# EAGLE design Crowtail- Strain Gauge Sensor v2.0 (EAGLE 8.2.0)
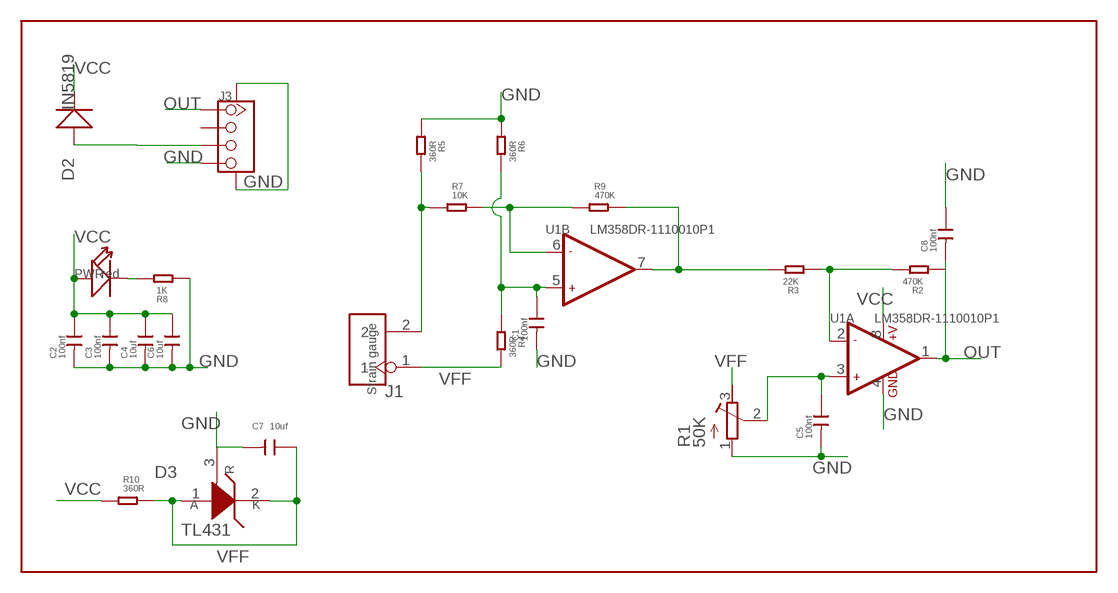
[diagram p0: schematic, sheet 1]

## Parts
C1  100nf  C-0603  [C0603]
C2  100nf  C-0603  [C0603]
C3  100nf  C-0603  [C0603]
C4  10uf  C-0603  [C0603]
C5  100nf  C-0603  [C0603]
C6  10uf  C-0603  [C0603]
C7  10uf  C-0603  [C0603]
C8  100nf  C-0603  [C0603]
D2  IN5819  D'0805'  [SOD323]
D3  TL431  [SOT23]
J1  Strain gauge  HEADER-2P-65/35MIL  [2P-2.54-65/35MIL]
J3  TWIG-4P-2.0-SMD-FEMALE-REINFORCE'90D'  [4P-SMD-2.0-90D]
PWR  red  LED'0603'  [LED-0603]
R1  50K  R-TRIMM3296P  [RTRIM3296P]
R2  470K  R-0603  [R0603]
R3  22K  R-0603  [R0603]
R4  360R  R-0603  [R0603]
R5  360R  R-0603  [R0603]
R6  360R  R-0603  [R0603]
R7  10K  R-0603  [R0603]
R8  1K  R-0603  [R0603]
R9  470K  R-0603  [R0603]
R10  360R  R-0603  [R0603]
U1  LM358DR-1110010P1  [SOIC8]

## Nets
GND: C1.2 C2.2 C3.2 C4.2 C5.2 C6.2 C7.2 C8.1 D3.3(R) J3.4 J3.SS1 J3.SS2 R1.1(E) R5.1 R6.1 R8.1 U1.4(A:GND)
N$1: C5.1 R1.2(S) U1.3(A:+IN1)
N$2: R2.2 R3.1 U1.2(A:-IN1)
N$3: R3.2 R9.2 U1.7(B:OUT2)
N$5: R7.2 R9.1 U1.6(B:-IN2)
N$6: J1.2 R5.2 R7.1
N$7: C1.1 R4.1 R6.2 U1.5(B:+IN2)
N$8: PWR.- R8.2
N$9: D2.+ J3.3
OUT: C8.2 J3.1 R2.1 U1.1(A:OUT1)
VCC: C2.1 C3.1 C4.1 C6.1 D2.- PWR.+ R10.1 U1.8(A:+V)
VFF: C7.1 D3.1(A) D3.2(K) J1.1 R1.3(A) R4.2 R10.2
Unconnected: J3.2

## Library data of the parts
C1-C8 = Discrete:C*: Ceramic Capacitors
D2 = Discrete:D*
D3 = Discrete:TL431
J1 = Connector:HEADER-2P
J3 = Connector:TWIG-4P-2.0-SMD-FEMALE-REINFORCE
PWR = Discrete:LED*
R1 = resistor:R-TRIMM: Trimm resistor
R2-R10 = Discrete:R*
U1 = OPL Eagle Library:LM358DR: General purpose LOW Voltage, Rail-to-Rail Output Amplifiers http://www.fairchildsemi.com/ds/LM/LMV358.pdf

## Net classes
3 usbvcc: width 0.203 mm, drill 0.305 mm, clearance 0.203 mm

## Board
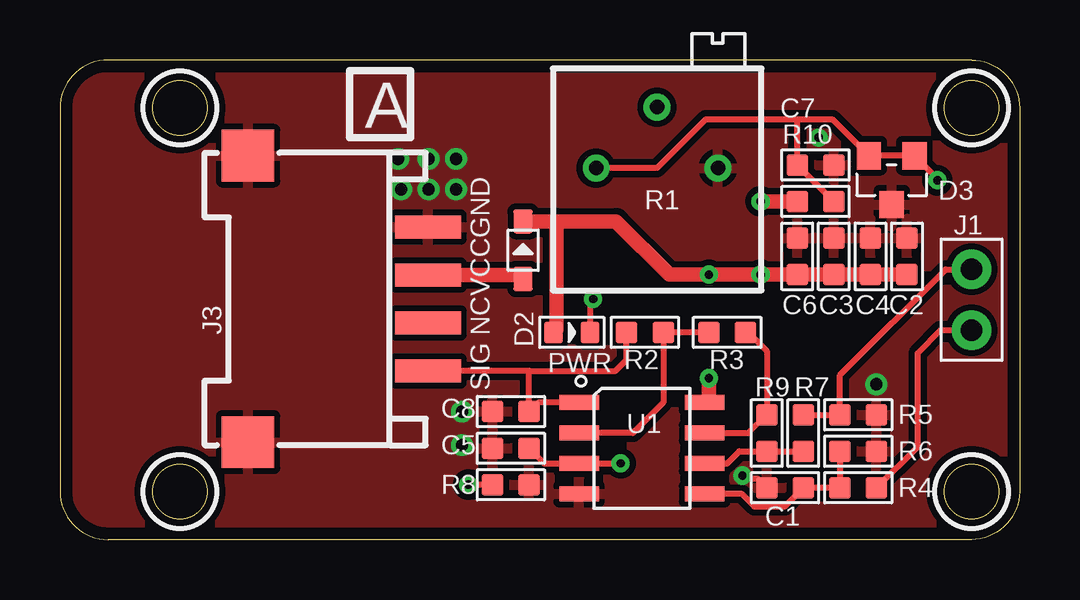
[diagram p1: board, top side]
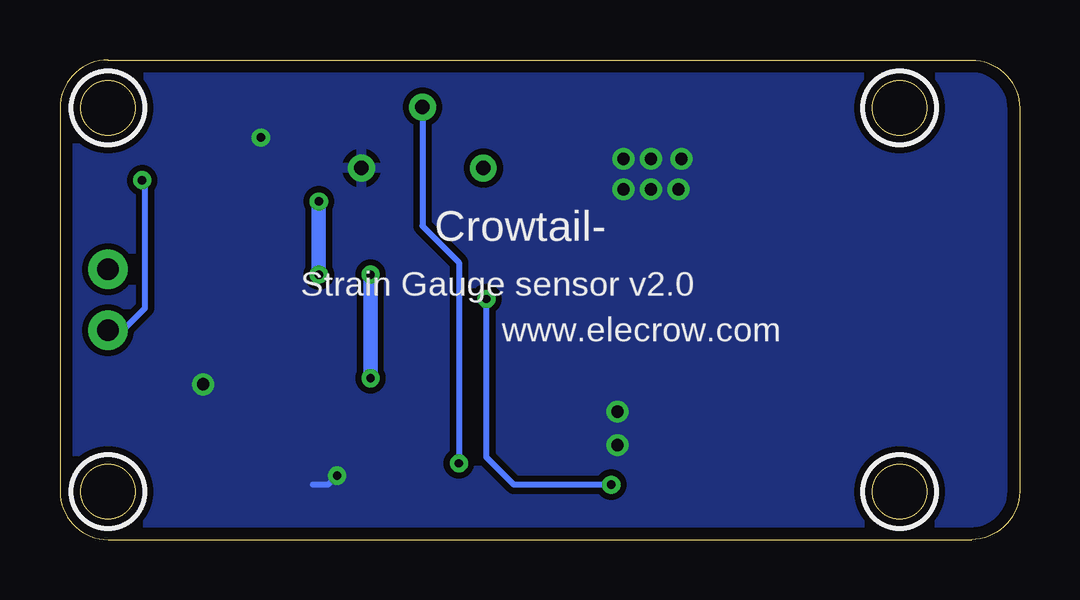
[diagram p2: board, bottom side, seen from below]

Size 40 x 20 mm. Coordinates in mm from the lower left corner, seen from the top.
Outline: 38,20 2,20 arc90 0,18 0,2 arc90 2,0 38,0 arc90 40,2 40,18 arc90 38,20
Outline: circle at 5,18 radius 1.14
Outline: circle at 5,2 radius 1.14
Outline: circle at 38,18 radius 1.14
Outline: circle at 38,2 radius 1.14
Copper layers (1*16): Top 0.035mm / dielectric 1.5mm / Bottom 0.035mm
Design rules "default *": minimum track width 10mil, minimum drill 20mil, track to track 8mil, track to pad 8mil, pad to pad 8mil, via to via 8mil, smd to smd 8mil, copper to edge 20mil, drill to drill 8mil, minimum pad ring 10mil, minimum via ring 8mil, stop-mask expansion 2mil, vias tented up to drill 100mil, thermal gap 10mil
tRestrict: area 3.5,16.5 to 6.5,19.5; area 3.5,0.5 to 6.5,3.5; area 36.5,16.5 to 39.5,19.5; area 36.5,0.5 to 39.5,3.5
bRestrict: area 3.5,16.5 to 6.5,19.5; area 3.5,0.5 to 6.5,3.5; area 36.5,16.5 to 39.5,19.5; area 36.5,0.5 to 39.5,3.5

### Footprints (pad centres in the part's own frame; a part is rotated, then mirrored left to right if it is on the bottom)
C0603 = smd 0.889 x 0.889: 1 -0.762,0; 2 0.762,0
SOD323 = smd 1 x 0.8: + -1.2,0; - 1.2,0
SOT23 = smd 1.016 x 1.143: 1 -0.95,-1.016; 2 0.95,-1.016; 3 0,1.016
2P-2.54-65/35MIL = drill 0.889 pad 1.651: 1 0,1.27; 2 0,-1.27
4P-SMD-2.0-90D = smd 0.965 x 2.74: 1 -3,-0.1; 2 -1,-0.1; 3 1,-0.1; 4 3,-0.1 | smd 2.159 x 2.184: SS1 -5.974,7.4; SS2 5.974,7.4
LED-0603 = smd 0.762 x 0.889: + -0.762,0; - 0.762,0
RTRIM3296P = drill 0.61: 1 0,-2.54; 2 2.54,0; 3 0,2.54
R0603 = smd 0.889 x 0.889: 1 -0.762,0; 2 0.762,0
SOIC8 = smd 1.651 x 0.635: 1 -2.616,1.905; 2 -2.616,0.635; 3 -2.616,-0.635; 4 -2.616,-1.905; 5 2.616,-1.905; 6 2.616,-0.635; 7 2.616,0.635; 8 2.616,1.905

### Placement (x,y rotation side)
C1  30.23,2.16 180 top
C2  35.31,11.81 90 top
C3  32.26,11.81 90 top
C4  33.78,11.81 90 top
C5  18.8,3.81 180 top
C6  30.73,11.81 90 top
C7  31.5,15.62 0 top
C8  18.8,5.33 0 top
D2  19.3,12.06 90 top
D3  34.67,14.99 180 top
J1  38,10 180 top
J3  15.24,10.03 90 top
PWR  21.34,8.64 0 top
R1  24.89,15.49 90 top
R2  24.38,8.64 0 top
R3  27.81,8.64 0 top
R4  33.27,2.16 0 top
R5  33.27,5.21 180 top
R6  33.27,3.68 180 top
R7  30.99,4.45 270 top
R8  18.8,2.29 180 top
R9  29.46,4.45 90 top
R10  31.5,14.1 0 top
U1  24.26,3.81 0 top

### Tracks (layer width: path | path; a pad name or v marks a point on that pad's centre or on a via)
GND  (via drill 0.35, 0.51)
  Top 0.254: C1.2 29.08,2.54 28.57,2.54 v28.45,2.67
  Bottom 0.254: v28.45,2.67 28.83,2.29 29.46,2.29
  other vias: 34.04,6.48 31.62,16.76 14.22,14.61 15.37,14.61 16.51,14.61 14.1,15.88 15.37,15.88 16.51,15.88 16.76,5.33 16.76,3.94
  pour Top (isolate 0.254): -1.27,20.32 41.91,20.32 41.91,0.05 arc-90 41.86,0 -1.27,0
  pour Bottom (isolate 0.254): -1.27,20.32 41.91,20.32 41.91,0 -1.27,0
N$1  (via drill 0.35)
  Top 0.254: C5.1 20.19,3.17 U1.3 v23.37,3.17
  Bottom 0.254: v23.37,3.17 23.37,11.56 24.89,13.08 R1.2
N$2
  Top 0.254: R3.1 R2.2 25.15,5.71 23.88,4.45 U1.2
N$3
  Top 0.254: U1.7 28.7,4.45 R9.2 29.46,7.87 28.7,8.64 R3.2
  Top 0.406: 29.34,4.95 R9.2
N$5
  Top 0.254: R7.2 R9.1 28.32,3.68 27.81,3.17 U1.6
N$6
  Top 0.254: R7.1 32.26,5.21 | J1.2 36.92,11.27 32.51,6.86 R5.2
  Top 0.406: 32.26,5.21 R5.2
N$7
  Top 0.254: U1.5 28.43,1.91 28.95,1.38 30.21,1.38 C1.1 R4.1 R6.2
N$8  (via drill 0.35)
  Top 0.254: R8.2 v17.02,2.29 | v22.23,10.03 22.1,9.91 PWR.-
  Bottom 0.254: v17.02,2.29 21.08,2.29 22.23,3.43 v22.23,10.03
N$9
  Top 0.61: J3.3 19.14,11.03 D2.+
OUT
  Top 0.254: 19.56,7.03 J3.1 | 19.56,7.03 23.16,7.03 23.62,7.49 R2.1 | U1.1 19.94,5.71 C8.2 19.56,7.03
VCC  (via drill 0.35)
  Top 0.406: C2.1 C4.1 C3.1 C6.1
  Top 0.61: 20.7,13.27 D2.- | 20.7,13.27 23.18,13.27 25.4,11.05 v27.05,11.05 v29.21,11.05 C2.1 | PWR.+ 20.7,8.76 20.7,13.27 | U1.8 27.05,5.89 v27.05,6.73 | R10.1 v29.21,14.1
  Bottom 0.61: v27.05,6.73 v27.05,11.05 | v29.21,14.1 v29.21,11.05
VFF  (via drill 0.35)
  Top 0.254: R4.2 35.75,3.87 35.75,7.78 36.7,8.73 J1.1 | R10.2 C7.1 30.73,17.53 | R1.3 24.89,15.49 26.92,17.53 30.73,17.53 | 30.73,17.53 32.2,17.53 D3.2 D3.1 36.58,15.05 v36.58,14.99
  Bottom 0.254: J1.1 37.37,8.73 36.45,9.65 36.45,14.86 v36.58,14.99

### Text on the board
tPlace: A | GND | VCC | NC | SIG
bPlace: Crowtail- | Strain Gauge sensor v2.0 | www.elecrow.com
